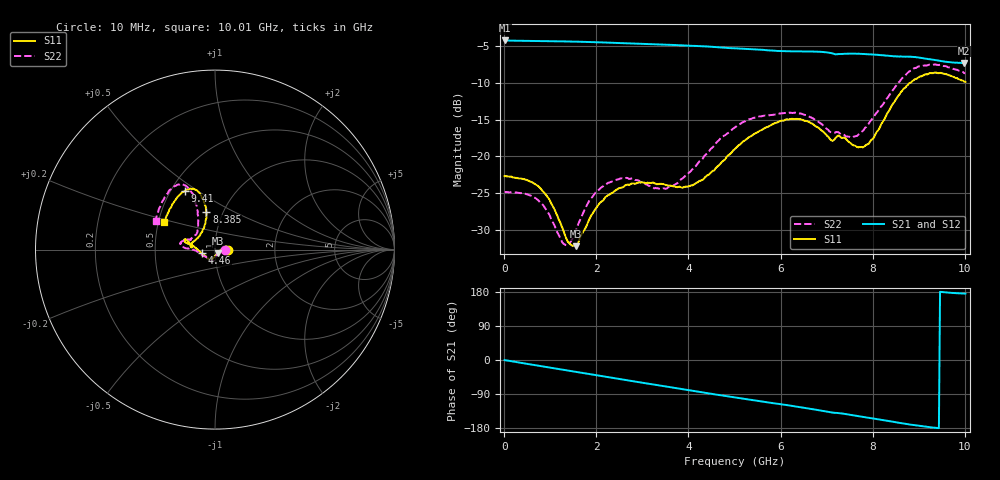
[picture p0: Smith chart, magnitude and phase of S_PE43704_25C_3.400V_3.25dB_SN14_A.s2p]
! Device ID: PE43704
! Dir: z:\PE43704\PE43704_Char_1_20130516\PE43704\AMB\3p400V\3p25dB
! Serial: 14
! Insertion: A
! Impedance: 50 ohm
! Temp: Amb
! VDD: 3.400V
! Attenuation Step: 3.25dB
! IDD: 1.140877e-01mA
#  Hz  S  RI  R  50
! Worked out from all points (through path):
!   401 points, 10 MHz to 10.01 GHz, reference 50 ohm
!   highest |S21| = -4.29 dB at 10 MHz (marker M1); lowest = -7.4 dB at 9.985 GHz (marker M2)
!   group delay of S21, straight-line fit = 52.6 ps
!   lowest |S11| = -32.2 dB at 1.56 GHz (marker M3), VSWR 1.05, Z = 51.4 - j2.07 ohm
!   |S11| at or under -10 dB: start of sweep to 8.818 GHz
!   |S22| runs from -32.1 to -7.5 dB; largest |S21 - S12| = 0.0038
!   S11 on the Smith chart (normalised r, x): 10 MHz: 1.16, +0.00; 4.46 GHz: 0.86, -0.04; 8.385 GHz: 0.84, +0.36; 9.41 GHz: 0.59, +0.44; 10.01 GHz: 0.54, +0.18
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1e7  0.0735 0.000194  0.6105 -0.0026  0.6107 -0.00233  0.0573 0.000269
7.6e8  0.0592 0.0185  0.5829 -0.1609  0.5829 -0.1608  0.0468 0.0164
1.31e9  0.0295 -0.00461  0.538 -0.2683  0.5381 -0.2682  0.023 -0.0108
1.56e9  0.0142 -0.0202  0.5108 -0.3131  0.5107 -0.3132  0.0114 -0.0294
1.685e9  0.00713 -0.0289  0.4954 -0.3348  0.4955 -0.3347  0.00566 -0.039
1.985e9  -0.00696 -0.0437  0.4546 -0.382  0.4547 -0.382  -0.00422 -0.0569
2.385e9  -0.0195 -0.0544  0.3939 -0.4369  0.3941 -0.4368  -0.0151 -0.0671
3.36e9  -0.0302 -0.0577  0.2244 -0.5278  0.225 -0.5275  -0.029 -0.053
3.985e9  -0.0479 -0.0401  0.1056 -0.5536  0.1061 -0.5533  -0.0695 -0.0319
4.46e9  -0.0734 -0.0209  0.0147 -0.5542  0.0154 -0.5545  -0.1099 -0.00417
5.01e9  -0.1117 0.0127  -0.0828 -0.5336  -0.0826 -0.5337  -0.1573 0.00665
5.985e9  -0.1638 0.0572  -0.2306 -0.464  -0.2282 -0.4645  -0.193 0.0311
6.685e9  -0.1624 0.0385  -0.3275 -0.3959  -0.328 -0.3952  -0.1752 0.0499
7.11e9  -0.1262 0.0207  -0.3741 -0.3321  -0.3749 -0.3326  -0.1358 0.0532
7.46e9  -0.1184 0.0458  -0.4003 -0.2948  -0.4003 -0.2951  -0.1102 0.0801
7.76e9  -0.088 0.0756  -0.4268 -0.2497  -0.4264 -0.2508  -0.0961 0.1109
8.36e9  -0.0477 0.2003  -0.4543 -0.1543  -0.4535 -0.1561  -0.1018 0.2398
8.385e9  -0.0476 0.2078  -0.4555 -0.1494  -0.4534 -0.152  -0.1024 0.2476
8.86e9  -0.0853 0.3129  -0.4671 -0.0724  -0.4642 -0.0734  -0.1602 0.3542
9.41e9  -0.1697 0.3252  -0.4466 -0.00314  -0.4466 -0.00187  -0.2406 0.3401
9.985e9  -0.2767 0.1629  -0.4275 0.0358  -0.4285 0.0371  -0.327 0.1663
1.001e10  -0.2818 0.1516  -0.4286 0.0366  -0.4306 0.0371  -0.3302 0.1575
